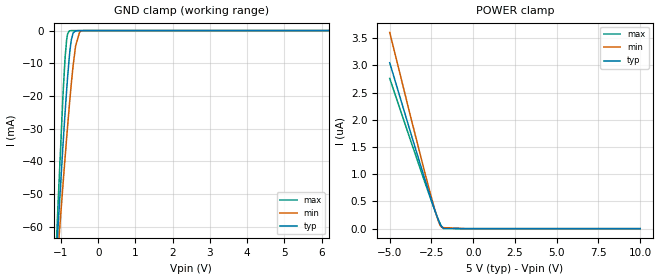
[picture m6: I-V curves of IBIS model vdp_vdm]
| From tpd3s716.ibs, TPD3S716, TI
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|   vdp_vdm Model
[Model]   vdp_vdm
Model_type   Terminator
|   typ   min   max
|   (nom PVT)   (fast PVT)   (slow PVT)
C_comp   1.437e-12   1.417e-12   1.619e-12
| Where nom  PVT is Nominal Process, 5V, 40C
|   Fast PVT is Strong Process,  5.5V, -40C
|   Slow PVT is Weak Process,   4.5V, 125C
[Voltage Range]   5   4.5   5.5
|Junction Temperature
[Temperature Range]   40   125   -40
[Power Clamp Reference]   5   4.5   5.5
[GND Clamp Reference]   0   0   0
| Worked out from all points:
|   GND clamp passes 1 mA (typ) near -0.68 V on its own axis
[GND Clamp]
|   Voltage   I(typ)   I(min)   I(max)
-5V       -889.8mA   -719.9mA   -1.198A
-1.11V    -66.25mA   -72.04mA   -61.52mA
-1.079V   -60.07mA   -67.16mA   -53.07mA
-945.5mV  -34.98mA   -47.01mA   -19.76mA
-891.5mV  -25.46mA   -39.1mA    -8.761mA
-846.5mV  -18.04mA   -32.67mA   -2.664mA
-760mV    -6.228mA   -20.96mA   -56.5uA
-675mV    -751.1uA   -10.85mA   -854.1nA
-608mV    -73.18uA   -4.74mA    -31.66nA
-500mV    -1.364uA   -465.2uA   0A
-428mV    -99.57nA   -62.48uA   0A
10V       0A         0A         0A
[POWER Clamp]
|   Voltage   I(typ)   I(min)   I(max)
-5V       3.048uA    3.605uA    2.759uA
-3.663V   1.679uA    1.954uA    1.543uA
-2.619V   638.3nA    706.4nA    610.4nA
-2.15V    209.3nA    199.8nA    215.4nA
-2.01V    103.1nA    81.62nA    111.6nA
-1.895V   39.04nA    28.33nA    44.27nA
-1.755V   0A         18.1nA     12.02nA
-500mV    0A         0A         0A
10V       0A         0A         0A
